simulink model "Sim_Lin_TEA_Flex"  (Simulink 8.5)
settings: Solver=ode23  StartTime=0.0  StopTime=108000  MaxStep=1  RelTol=1e-3
InitFcn:
  | start
StopFcn:
  | pl2
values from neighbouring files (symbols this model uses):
  Kpqr = lqr(sys,Q0,R0)    [des.m]
  wo = 0.0011    [start.m]    (also in start1.m; start2.m; start3.m)
undefined symbols (not defined in the file or in its folder): Af, Bf, Cf, Df

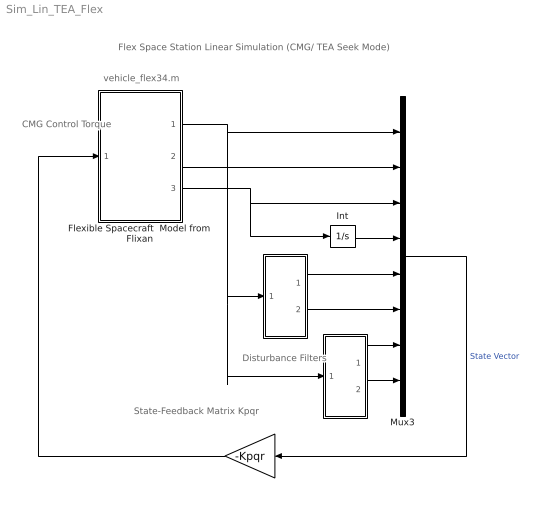
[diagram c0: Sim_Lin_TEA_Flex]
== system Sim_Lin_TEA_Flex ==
  note: Flex Space Station Linear Simulation (CMG/ TEA Seek Mode)
  note: State-Feedback Matrix Kpqr
  note: CMG Control Torque
  note: Disturbance Filters
  note: vehicle_flex34.m
  " " : Gain  Gain=-Kpqr  Multiplication=Matrix(K*u)
  "  " : Subsystem
  "    " : Subsystem
  Flexible Spacecraft  Model from Flixan : Subsystem
  Int : Integrator
  Mux3 : Mux  Inputs=[3, 3, 3, 3, 1, 1, 1, 1]
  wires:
  Int/1 -> Mux3/4
  Mux3/1 -> " "/1  "State Vector"
  "  "/1(a1) -> Mux3/5
  "  "/2(a2) -> Mux3/6
  Flexible Spacecraft  Model from Flixan/3("Hcmg ") -> Int/1, Mux3/3
  " "/1 -> Flexible Spacecraft  Model from Flixan/1(Tcmg)
  Flexible Spacecraft  Model from Flixan/1(att-lv) -> "    "/1(psi), "  "/1(the), Mux3/1
  Flexible Spacecraft  Model from Flixan/2(w-lv) -> Mux3/2
  "    "/1(b1) -> Mux3/7
  "    "/2(b2) -> Mux3/8

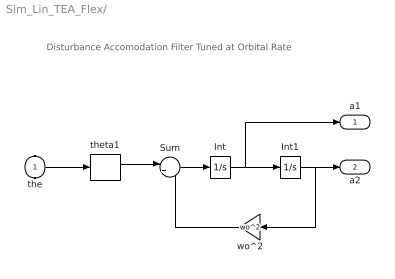
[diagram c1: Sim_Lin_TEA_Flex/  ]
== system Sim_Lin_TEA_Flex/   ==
  note: Disturbance Accomodation Filter Tuned at Orbital Rate
  the : Inport
  Int : Integrator
  Int1 : Integrator
  Sum : Sum  Inputs=|+-
  theta1 : Selector  InputPortWidth=3  Indices=[2]
  wo^2 : Gain  Gain=wo^2
  a1 : Outport
  a2 : Outport  Port=2
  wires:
  Int/1 -> Int1/1, a1/1
  Sum/1 -> Int/1
  Int1/1 -> wo^2/1, a2/1
  wo^2/1 -> Sum/2
  theta1/1 -> Sum/1
  the/1 -> theta1/1

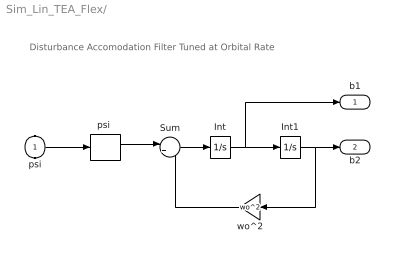
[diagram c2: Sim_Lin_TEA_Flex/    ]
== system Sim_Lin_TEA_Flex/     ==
  note: Disturbance Accomodation Filter Tuned at Orbital Rate
  psi : Inport
  Int : Integrator
  Int1 : Integrator
  Sum : Sum  Inputs=|+-
  "psi " : Selector  InputPortWidth=3  Indices=[3]
  wo^2 : Gain  Gain=wo^2
  b1 : Outport
  b2 : Outport  Port=2
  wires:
  Int/1 -> Int1/1, b1/1
  Sum/1 -> Int/1
  Int1/1 -> wo^2/1, b2/1
  wo^2/1 -> Sum/2
  "psi "/1 -> Sum/1
  psi/1 -> "psi "/1

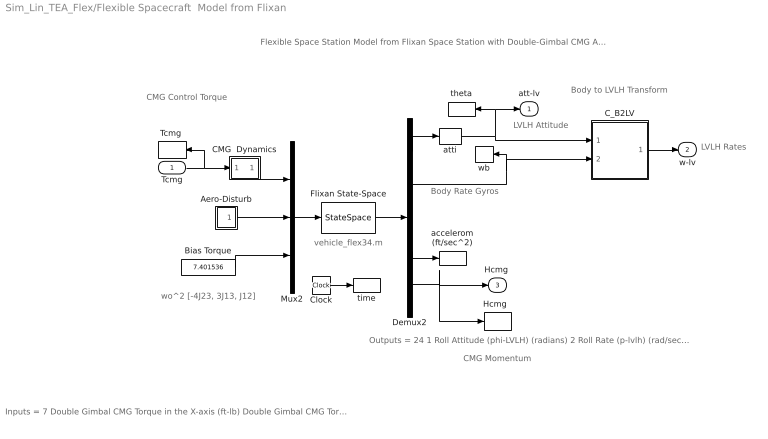
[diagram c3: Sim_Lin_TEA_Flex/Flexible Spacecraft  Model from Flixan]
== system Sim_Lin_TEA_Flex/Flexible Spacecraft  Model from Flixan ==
  note: vehicle_flex34.m
  note: Body to LVLH Transform
  note: LVLH Attitude
  note: Body Rate Gyros
  note: Flexible Space Station Model from Flixan Space Station with Double-Gimbal CMG Array (Flex)
  note: Inputs = 7 Double Gimbal CMG Torque in the X-axis (ft-lb) Double Gimbal CMG Torque in the Y-axis (ft-lb) Double Gimbal CMG Torque in the Z-axis (ft-lb) External Torque Input 1 (ft-lb), direct: External Torque Input 2 (ft-lb), direct: External Torque Input 3 (ft-lb), direct: Ext Torque Direct.=(0.197, -0.5964, -0.7782)
  note: Outputs = 24 1 Roll Attitude (phi-LVLH) (radians) 2 Roll Rate (p-lvlh) (rad/sec) 3 Pitch Attitude (thet-LVLH) (radians) 4 Pitch Rate (q-lvlh) (rad/sec) 5 Yaw Attitude (psi-LVLH) (radians) 6 Yaw Rate (r-lvlh) (rad/sec) 7 Angle of attack, alfa, (radians) 8 Angle of sideslip, beta, (radian) 9 Change in Altitude, delta-h, (feet) 10 Forward Acceleration (V-dot) (ft/sec) 11 Cross Range Velocity (Vcr) (ft/sec) 12 Rate-Gyro # 1, Roll Rate (Body) (rad/sec) 13 Rate-Gyro # 2, Pitch Rate (Body) (rad/sec) 14 Rate-Gyro # 3, Yaw Rate (Body) (rad/sec) 15 Gyro # 4, Roll Attitude (Body) (radians) 16 Gyro # 5, Pitch Attitude (Body) (radians) 17 Gyro # 6, Yaw Attitude (Body) (radians) 18 Accelerom # 1, (along X), (ft/sec^2) Translat. Accelerat. 19 Accelerom # 2, (along Z), (ft/sec^2) Translat. Accelerat. 20 Accelerom # 3, (along X), (ft/sec^2) Translat. Accelerat. 21 Accelerom # 4, (along Z), (ft/sec^2) Translat. Accelerat. 22 Double Gimbal CMG Momentum Change in X-axis (ft-lb-sec) 23 Double Gimbal CMG Momentum Change in Y-axis (ft-lb-sec) 24 Double Gimbal CMG Momentum Change in Z-axis (ft-lb-sec)
  note: CMG Control Torque
  note: LVLH Rates
  note: CMG Momentum
  note: wo^2 [-4J23, 3J13, J12]
  Tcmg : Inport  PortDimensions=3
  Aero-Disturb : Subsystem
  Bias Torque : Constant  Value=7.401536
  CMG  Dynamics : Subsystem
  C_B2LV : Subsystem
  Clock : Clock
  Demux2 : Demux  Outputs=[11, 3, 3, 4, 3]
  Flixan State-Space : StateSpace  A=Af  B=Bf  C=Cf  D=Df  X0=0
  "Hcmg  " : ToWorkspace  VariableName=Hcmg  SampleTime=-1
  Mux2 : Mux  Inputs=[3, 3, 1]
  "Tcmg " : ToWorkspace  VariableName=Tcmg  SampleTime=-1
  accelerom (ft/sec^2) : ToWorkspace  VariableName=accel  SampleTime=-1
  atti : Selector  InputPortWidth=11  Indices=[1 3 5]
  theta : ToWorkspace  VariableName=theta  SampleTime=-1
  time : ToWorkspace  VariableName=time  SampleTime=-1
  wb : ToWorkspace  VariableName=wb  SampleTime=-1
  att-lv : Outport
  w-lv : Outport  Port=2
  "Hcmg " : Outport  Port=3
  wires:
  Demux2/2 -> C_B2LV/2(wb), wb/1
  C_B2LV/1(wlv) -> w-lv/1
  atti/1 -> C_B2LV/1(atti), att-lv/1, theta/1
  CMG  Dynamics/1(O) -> Mux2/1
  Aero-Disturb/1(Td) -> Mux2/2
  Tcmg/1 -> "Tcmg "/1, CMG  Dynamics/1(I)
  Demux2/4 -> accelerom (ft/sec^2)/1
  Demux2/1 -> atti/1
  Demux2/5 -> "Hcmg "/1, "Hcmg  "/1
  Clock/1 -> time/1
  Bias Torque/1 -> Mux2/3
  Flixan State-Space/1 -> Demux2/1
  Mux2/1 -> Flixan State-Space/1

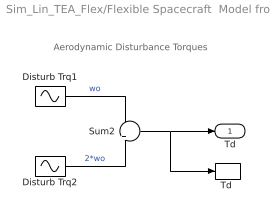
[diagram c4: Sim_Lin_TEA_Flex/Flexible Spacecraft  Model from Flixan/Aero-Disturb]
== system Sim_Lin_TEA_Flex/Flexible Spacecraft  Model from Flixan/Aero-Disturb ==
  note: Aerodynamic Disturbance Torques
  Disturb Trq1 : Sin  Amplitude=[1, 3, 1]  Bias="[1  8  1]"  Frequency=[wo, wo, wo]  SampleTime=0
  Disturb Trq2 : Sin  Amplitude=[1, 1, 1]*0.5  Frequency=[wo, wo, wo]*2  SampleTime=0
  Sum2 : Sum  Inputs=+|+
  "Td " : ToWorkspace  VariableName=Td  SampleTime=-1
  Td : Outport
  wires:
  Disturb Trq2/1 -> Sum2/2  "2*wo"
  Sum2/1 -> "Td "/1, Td/1
  Disturb Trq1/1 -> Sum2/1  "wo"

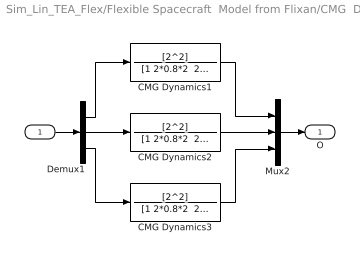
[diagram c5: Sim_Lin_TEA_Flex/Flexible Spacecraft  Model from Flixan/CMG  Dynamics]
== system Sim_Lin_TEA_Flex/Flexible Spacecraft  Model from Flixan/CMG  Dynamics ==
  I : Inport
  CMG Dynamics1 : TransferFcn  Numerator=[2^2]  Denominator="[1 2*0.8*2  2^2]"
  CMG Dynamics2 : TransferFcn  Numerator=[2^2]  Denominator="[1 2*0.8*2  2^2]"
  CMG Dynamics3 : TransferFcn  Numerator=[2^2]  Denominator="[1 2*0.8*2  2^2]"
  Demux1 : Demux  Outputs=3
  Mux2 : Mux  Inputs=3
  O : Outport
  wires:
  CMG Dynamics2/1 -> Mux2/2
  CMG Dynamics3/1 -> Mux2/3
  CMG Dynamics1/1 -> Mux2/1
  Demux1/2 -> CMG Dynamics2/1
  Demux1/1 -> CMG Dynamics1/1
  Demux1/3 -> CMG Dynamics3/1
  I/1 -> Demux1/1
  Mux2/1 -> O/1

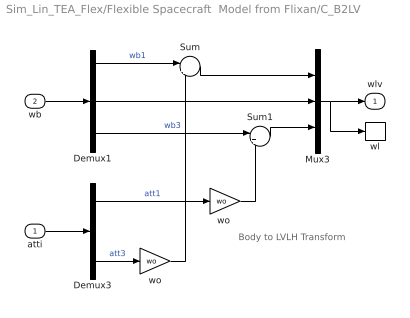
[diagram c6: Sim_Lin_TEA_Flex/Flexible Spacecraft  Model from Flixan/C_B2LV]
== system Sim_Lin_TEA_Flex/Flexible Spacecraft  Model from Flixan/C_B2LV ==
  note: Body to LVLH Transform
  atti : Inport  PortDimensions=3
  wb : Inport  Port=2  PortDimensions=3
  Demux1 : Demux  Outputs=3
  Demux3 : Demux  Outputs=3
  Mux3 : Mux  Inputs=3
  Sum : Sum  Inputs=|++
  Sum1 : Sum  Inputs=|+-
  wl : ToWorkspace  VariableName=wl  SampleTime=-1
  wo : Gain  Gain=wo
  "wo " : Gain  Gain=wo
  wlv : Outport
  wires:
  Demux1/1 -> Sum/1  "wb1"
  Sum/1 -> Mux3/1
  Demux3/3 -> wo/1  "att3"
  Sum1/1 -> Mux3/3
  atti/1 -> Demux3/1
  wb/1 -> Demux1/1
  Mux3/1 -> wlv/1, wl/1
  Demux3/1 -> "wo "/1  "att1"
  Demux1/2 -> Mux3/2
  wo/1 -> Sum/2
  Demux1/3 -> Sum1/1  "wb3"
  "wo "/1 -> Sum1/2
